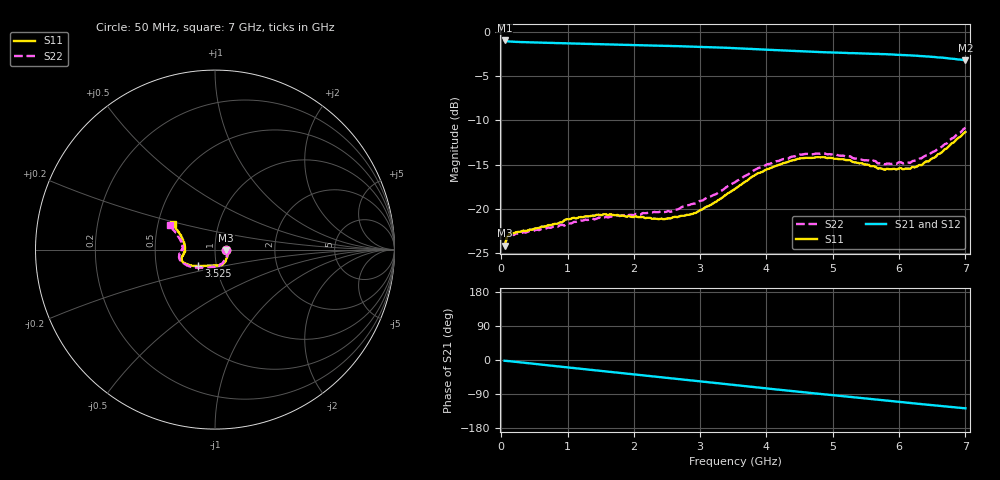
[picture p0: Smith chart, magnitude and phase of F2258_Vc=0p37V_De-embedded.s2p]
! Integrated Device Technology
! Corporate Headquarters
! 6024 Silver Creek Valley Road
! San Jose, CA 95138  USA
! Phone:  1-408-284-8200
! Toll Free:  1-800-223-1366
! Webpage:  http://www.idt.com/
! Timing and RF Division
! 515 Groton Road, Suite 102
! Westford, MA 01886-6024
! Device:  F2258
! Description: Voltage Variable RF Attenuator
! Frequency:  50.0 -  6000.00 MHz
! Package:  3x3 mm Thin QFN Plastic Package: 16 pin
! Ports:  2 RF, 2 DC
!  Pin  1  = NC
!  Pin  2  = NC
!  Pin  3  = RF2  = Port 2
!  Pin  4  = GND
!  Pin  5  = Vdd
!  Pin  6  = NC
!  Pin  7  = VCTRL
!  Pin  8  = NC
!  Pin  9  = GND
!  Pin 10  = RF1  = Port 1
!  Pin 11  = NC
!  Pin 12  = NC
!  Pin 13  = NC
!  Pin 14  = NC
!  Pin 15  = NC
!  Pin 16  = NC
! Vcntrl:  0.370 Volts
! Vdd:  +3.300 Volts
! Current:  1.092 mA
! Data:  The device was measured on a the F2258 evaluation board which has
!  individual transmission lines to the RF pins.  Data was collected
!  using a calibrated network analyzer.  The evaluation board was
!  de-embedded using a TRL calibration technique.
!  The reference plane is the edge of the package pin.
! Misc:  SN 10
!  Action Tracker AT0285
! Date Measured:  2014-12-10
! Date:  2016-01-13  MJV
! Note:
!  Integrated Device Technology supplies this data as a sample of measured
!  data at the package pin for this product.  Your particular data for this
!  product may vary.
!  Data was taken at 25 degrees C.
!  Integrated Device Technology reserves the right to change this data at anytime.
!Freq_(GHz)  S11M_(dB)  S11P_(deg)  S21M_(dB)  S21P_(deg)  S12M_(dB)  S12P_(deg)  S22M_(dB)  S22P_(deg)
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# GHz S dB R 50
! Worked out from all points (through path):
!   201 points, 50 MHz to 7 GHz, reference 50 ohm
!   highest |S21| = -1.01 dB at 50 MHz (marker M1); lowest = -3.2 dB at 7 GHz (marker M2)
!   group delay of S21, straight-line fit = 50.5 ps
!   lowest |S11| = -24.1 dB at 50 MHz (marker M3), VSWR 1.13, Z = 56.6 - j0.41 ohm
!   |S11| at or under -10 dB: start of sweep to end of sweep
!   |S22| runs from -24.2 to -10.8 dB; largest |S21 - S12| = 0.00049
!   S11 on the Smith chart (normalised r, x): 50 MHz: 1.13, -0.01; 3.525 GHz: 0.82, -0.15; 7 GHz: 0.60, +0.18
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0.05  -24.13 -3.3  -1.01 -1.9  -1.01 -1.9  -24.20 -3.0
0.08475  -23.18 -5.6  -1.08 -2.5  -1.08 -2.5  -23.28 -5.3
0.15425  -22.72 -8.7  -1.14 -3.6  -1.14 -3.6  -22.91 -9.1
0.71025  -21.82 -35.2  -1.27 -14.1  -1.27 -14.1  -22.10 -37.4
0.98825  -21.15 -48.6  -1.33 -19.4  -1.33 -19.4  -21.66 -53.1
1.2315  -20.94 -56.7  -1.38 -23.8  -1.38 -23.8  -21.31 -62.0
1.6485  -20.60 -68.2  -1.47 -31.4  -1.47 -31.4  -20.87 -75.1
2.37825  -21.15 -88.9  -1.59 -44.8  -1.60 -44.8  -20.35 -93.0
2.552  -21.08 -94.9  -1.63 -48.0  -1.63 -48.0  -20.33 -98.4
2.93425  -20.44 -111.6  -1.71 -55.1  -1.71 -55.1  -19.39 -111.8
3.247  -19.16 -124.5  -1.79 -61.0  -1.79 -61.0  -18.30 -124.1
3.525  -17.75 -135.2  -1.87 -66.2  -1.87 -66.2  -16.99 -134.7
4.0115  -15.51 -149.4  -2.05 -75.2  -2.05 -75.2  -14.96 -150.3
4.46325  -14.37 -158.1  -2.21 -83.4  -2.21 -83.4  -13.94 -161.5
4.7065  -14.23 -161.4  -2.28 -87.7  -2.29 -87.7  -13.83 -165.7
5.2625  -14.51 -168.2  -2.44 -97.4  -2.44 -97.4  -14.07 -173.9
5.6795  -15.45 -174.8  -2.52 -104.6  -2.52 -104.6  -14.86 -179.4
5.85325  -15.52 -179.0  -2.58 -107.8  -2.58 -107.8  -14.90 176.0
6.166  -15.47 173.1  -2.68 -113.4  -2.69 -113.4  -14.81 170.0
6.33975  -15.07 166.6  -2.77 -116.5  -2.77 -116.5  -14.28 165.6
6.722  -13.15 154.6  -3.00 -123.1  -3.00 -123.1  -12.61 156.6
7  -11.32 148.9  -3.24 -127.4  -3.25 -127.4  -10.84 151.6
